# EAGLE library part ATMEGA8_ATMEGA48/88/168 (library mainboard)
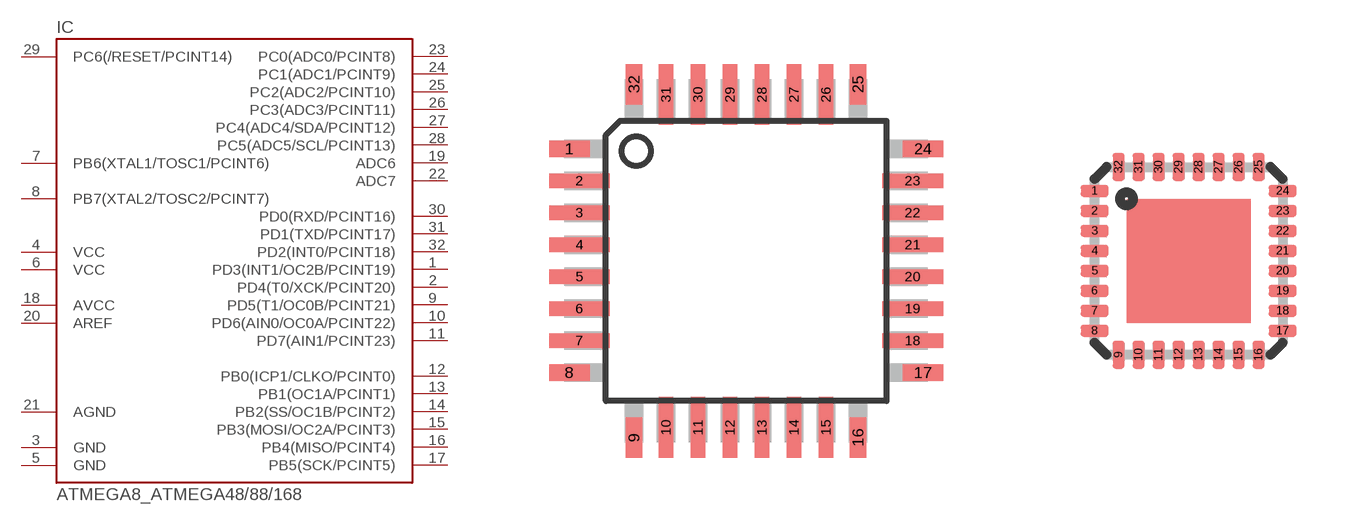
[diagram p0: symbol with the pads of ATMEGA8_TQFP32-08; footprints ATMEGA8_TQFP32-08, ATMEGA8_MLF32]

Designator prefix IC

## ATMEGA8_ATMEGA48/88/168-AU  [ATMEGA8_TQFP32-08]
1  PD3(INT1/OC2B/PCINT19)
2  PD4(T0/XCK/PCINT20)
3  GND  pwr
4  VCC  pwr
5  GND  pwr
6  VCC  pwr
7  PB6(XTAL1/TOSC1/PCINT6)
8  PB7(XTAL2/TOSC2/PCINT7)
9  PD5(T1/OC0B/PCINT21)
10  PD6(AIN0/OC0A/PCINT22)
11  PD7(AIN1/PCINT23)
12  PB0(ICP1/CLKO/PCINT0)
13  PB1(OC1A/PCINT1)
14  PB2(SS/OC1B/PCINT2)
15  PB3(MOSI/OC2A/PCINT3)
16  PB4(MISO/PCINT4)
17  PB5(SCK/PCINT5)
18  AVCC  pas
19  ADC6  pas
20  AREF  pas
21  AGND  pwr
22  ADC7  pas
23  PC0(ADC0/PCINT8)
24  PC1(ADC1/PCINT9)
25  PC2(ADC2/PCINT10)
26  PC3(ADC3/PCINT11)
27  PC4(ADC4/SDA/PCINT12)
28  PC5(ADC5/SCL/PCINT13)
29  PC6(/RESET/PCINT14)
30  PD0(RXD/PCINT16)
31  PD1(TXD/PCINT17)
32  PD2(INT0/PCINT18)

## ATMEGA8_ATMEGA48/88/168-MU  [ATMEGA8_MLF32]
Pads as for ATMEGA8_TQFP32-08

## Footprint ATMEGA8_TQFP32-08 (pad centres in mm)
Thin Plasic Quad Flat Package Grid 0.8 mm
smd 1.016 x 0.406: 1 -4.42,2.8; 8 -4.42,-2.8; 17 4.42,-2.8; 24 4.42,2.8
smd 1.524 x 0.356: 2 -4.166,2; 3 -4.166,1.2; 4 -4.166,0.4; 5 -4.166,-0.4; 6 -4.166,-1.2; 7 -4.166,-2; 18 4.166,-2; 19 4.166,-1.2; 20 4.166,-0.4; 21 4.166,0.4; 22 4.166,1.2; 23 4.166,2
smd 0.406 x 1.016: 9 -2.8,-4.42; 16 2.8,-4.42; 25 2.8,4.42; 32 -2.8,4.42
smd 0.356 x 1.524: 10 -2,-4.166; 11 -1.2,-4.166; 12 -0.4,-4.166; 13 0.4,-4.166; 14 1.2,-4.166; 15 2,-4.166; 26 2,4.166; 27 1.2,4.166; 28 0.4,4.166; 29 -0.4,4.166; 30 -1.2,4.166; 31 -2,4.166

## Footprint ATMEGA8_MLF32 (pad centres in mm)
32M1-A Micro Lead Frame package (MLF)
smd 0.7 x 0.3: 1 -2.35,1.75; 2 -2.35,1.25; 3 -2.35,0.75; 4 -2.35,0.25; 5 -2.35,-0.25; 6 -2.35,-0.75; 7 -2.35,-1.25; 8 -2.35,-1.75; 17 2.35,-1.75; 18 2.35,-1.25; 19 2.35,-0.75; 20 2.35,-0.25; 21 2.35,0.25; 22 2.35,0.75; 23 2.35,1.25; 24 2.35,1.75
smd 0.3 x 0.7: 9 -1.75,-2.35; 10 -1.25,-2.35; 11 -0.75,-2.35; 12 -0.25,-2.35; 13 0.25,-2.35; 14 0.75,-2.35; 15 1.25,-2.35; 16 1.75,-2.35; 25 1.75,2.35; 26 1.25,2.35; 27 0.75,2.35; 28 0.25,2.35; 29 -0.25,2.35; 30 -0.75,2.35; 31 -1.25,2.35; 32 -1.75,2.35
